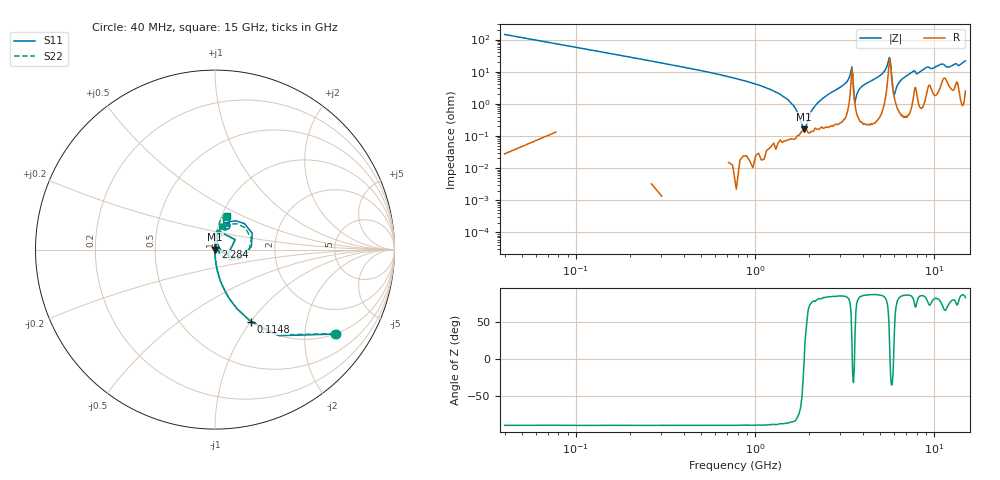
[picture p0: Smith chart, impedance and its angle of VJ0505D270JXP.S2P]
! VJ0505D270JXP
! MLCC placed on 25 mil thick microstrip substrate in series configuraton.
! DATE 06/29/2018  09:13
! CORRECTED  DATA
# GHz  S  MA  R  50.00
!  FREQ  S11M  S11A  S21M  S21A  S12M  S12A  S22M  S22A
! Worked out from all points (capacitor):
!   401 points, 40 MHz to 15 GHz, reference 50 ohm
!   read as one part in series: C = 27.7 pF near 114.8 MHz
!   lowest |Z| = 162 mohm at 1.873 GHz (marker M1)
!   series resonance near 1.886 GHz, so ESL is about 260 pH
!   S11 on the Smith chart (normalised r, x): 40 MHz: 0.99, -2.88; 114.8 MHz: 1.00, -1.00; 2.284 GHz: 1.00, +0.03; 15 GHz: 1.07, +0.41
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0.04  0.8228 -34.9  0.5712 55.1  0.5717 55.1  0.8155 -35.0
0.1148  0.4473 -63.7  0.894 26.5  0.8952 26.5  0.4432 -63.8
0.1896  0.2886 -73.5  0.9567 16.7  0.957 16.7  0.2862 -73.7
0.414  0.1316 -82.5  0.9901 7.5  0.9907 7.6  0.1306 -83.0
1.4612  0.01519 -87.0  0.998 0.9  0.9983 1.0  0.01515 -93.6
1.7978  0.002482 -61.4  0.9974 0.1  0.9981 0.3  0.002186 -111.0
1.8726  0.001439 17.4  0.9965 0.0  0.998 0.1  0.000817 134.7
2.0596  0.006774 77.6  0.9976 -0.3  0.9977 -0.2  0.006787 94.6
2.284  0.01282 81.3  0.997 -0.6  0.9976 -0.5  0.01294 92.3
2.5458  0.02035 83.7  0.9967 -1.0  0.9971 -0.9  0.02074 89.5
3.1816  0.04336 82.8  0.9944 -2.3  0.995 -2.2  0.04428 86.0
3.4434  0.1011 58.5  0.9506 -5.1  0.9508 -5.0  0.1015 60.4
3.6678  0.01687 66.4  0.9923 -0.7  0.9927 -0.6  0.01641 74.9
3.9296  0.03459 82.0  0.9954 -1.8  0.9959 -1.7  0.03414 88.2
5.0516  0.08045 82.4  0.9911 -4.4  0.9914 -4.3  0.07859 83.9
5.65  0.2265 23.8  0.7968 -5.2  0.7975 -5.2  0.2117 16.5
5.9866  0.02696 20.2  0.9814 -0.3  0.9819 -0.2  0.0102 39.7
6.4354  0.0511 75.3  0.992 -2.7  0.9929 -2.6  0.04956 90.4
7.52  0.0948 76.7  0.9864 -5.3  0.9872 -5.3  0.0948 84.2
10.0258  0.1294 72.5  0.9714 -7.4  0.9726 -7.4  0.1266 77.2
12.5316  0.1403 65.7  0.962 -8.5  0.9628 -8.6  0.1348 75.4
15  0.197 69.8  0.9547 -12.7  0.9554 -12.7  0.1928 71.8
